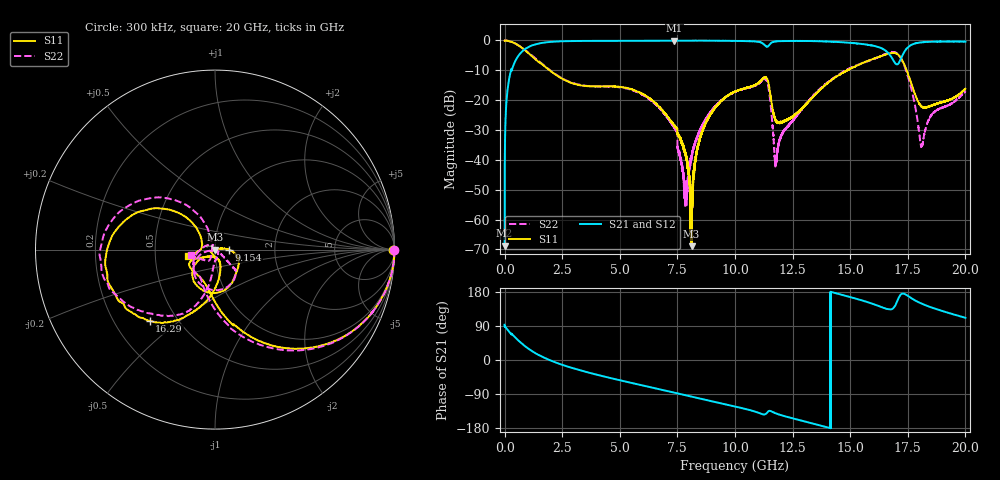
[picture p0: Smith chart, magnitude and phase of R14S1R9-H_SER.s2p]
!{R14S1R9}
!Johanson Technology Inc.
!www.johansontechnology.com
!Test Board Conditions:
!Substrate Type  RO4350B
!Substrate Thickness  20 mil
!Substrate Dk  3.66
!TL Type: GCPW
!TL Trace Width  36 mil
!TL Gap  12 mil
!Electrode orientation  Horizontal
!DUT TOPOLOGY	SERIES
!Mounting Pad LxW  26x36 mil
! Created Wed Nov 25 17:33:21 2020
! 2 Port Network Data from SP1.SP block
! freq  magS11  angS11  magS21  angS21  magS12  angS12  magS22  angS22
# khz S ma R 50
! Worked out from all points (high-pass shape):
!   20001 points, 300 kHz to 20 GHz, reference 50 ohm
!   highest |S21| = -0.04 dB at 7.367 GHz (marker M1); lowest = -68.8 dB at 300 kHz (marker M2)
!   |S21| within 3 dB of the highest: 860.1 MHz to 16.46 GHz (15.6 GHz wide, 180 % of centre); 17.42 GHz to end of sweep
!   lowest |S11| = -68.9 dB at 8.117 GHz (marker M3), VSWR 1.00, Z = 50 + j0.0357 ohm
!   |S11| at or under -10 dB: 1.954 GHz to 14.87 GHz (12.91 GHz wide, 154 % of centre); 14.86953 GHz to 14.87416 GHz (4.63 MHz wide, 0.0311 % of centre); 17.45 GHz to end of sweep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
!   |S22| runs from -56.0 to 0.0 dB; largest |S21 - S12| = 0.015
!   S11 on the Smith chart (normalised r, x): 300 kHz: open; 9.154 GHz: 1.17, -0.00; 16.29 GHz: 0.35, -0.39; 20 GHz: 0.74, -0.06
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300  0.9945 -0.1  0.0003649 93.0  0.0003593 81.3  0.9969 -0.1
133300  0.9868 -10.2  0.1562 79.6  0.1569 79.5  0.9869 -10.2
499300  0.8731 -33.0  0.4801 57.2  0.4816 57.3  0.8753 -33.0
1611300  0.4031 -79.1  0.9086 9.4  0.9086 9.4  0.4113 -81.7
3334300  0.1766 -117.2  0.9808 -28.0  0.9809 -28.0  0.1782 -116.7
6667300  0.08024 -147.3  0.9916 -76.5  0.9931 -76.5  0.07716 176.6
7367300  0.0379 -111.2  0.9959 -86.2  0.9944 -86.2  0.03411 126.5
7856300  0.01294 -158.0  0.9928 -93.0  0.994 -93.0  0.00308 -121.8
8117300  0.000359 96.5  0.9917 -96.7  0.9938 -96.7  0.01137 -38.5
8437300  0.0204 12.1  0.9938 -101.2  0.9919 -101.1  0.02862 -36.0
9154300  0.07639 -0.0  0.9886 -111.1  0.9899 -111.1  0.08034 -41.6
1.00003e7  0.1387 -21.2  0.9831 -122.8  0.9816 -122.8  0.1379 -44.3
1.13453e7  0.2411 -101.3  0.8018 -142.0  0.8013 -141.9  0.221 -101.0
1.17893e7  0.0443 -120.2  0.9659 -141.2  0.9663 -141.1  0.009754 -76.7
1.20893e7  0.04377 -89.9  0.9761 -147.1  0.9795 -147.1  0.02874 -53.7
1.33343e7  0.109 -73.7  0.9747 -167.0  0.9777 -167.0  0.1113 -96.1
1.62923e7  0.5381 -132.5  0.7596 141.1  0.7525 141.4  0.5406 -141.1
1.66673e7  0.5972 -150.1  0.6079 133.7  0.5951 133.6  0.626 -159.8
1.73683e7  0.3781 142.8  0.6619 174.0  0.659 174.4  0.3618 129.7
1.80993e7  0.07806 156.6  0.9302 148.8  0.9311 148.5  0.01744 -177.1
1.85833e7  0.08259 -177.4  0.9531 137.4  0.9502 137.5  0.06026 -116.6
2e7  0.1553 -165.9  0.9549 111.3  0.9542 111.6  0.1408 -167.1
